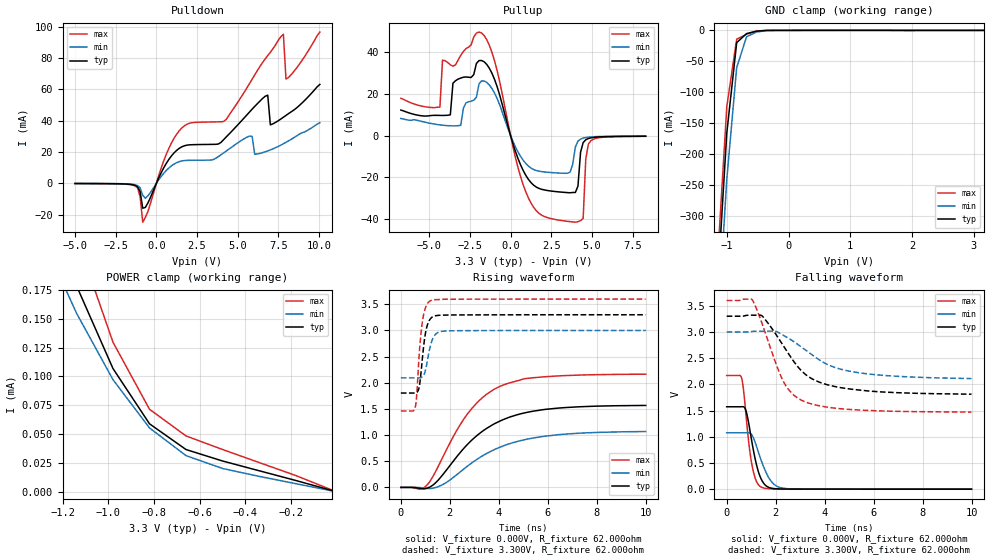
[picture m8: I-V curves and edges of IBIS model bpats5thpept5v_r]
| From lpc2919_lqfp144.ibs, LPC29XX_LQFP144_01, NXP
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| |   Rev 0.20 IBIS Model Design Automation Generation   |
| |   N O N - S I L I C O N   C O R R E L A T E D   |
| |   This IBIS [Model] is pre-Beta tactical support   |
| |  Note: this IBIS [Model] contains clamp curves generated   |
| |   through simulation which should not be relied upon   |
| Pccmos14 hliolib_nlm 4.0.1
|   0.18 um 3.3V pad library
|   six level metal
|   dual oxide
|   single threshold voltage
|   nominal line mixed supply
|   parasitic extracted netlists
| Process block c14
| bpats5thpept5v
|   Bidirectional Pad 3v3
|   3state Output
|   Plain Input
|   5ns Slew Rate control
|   CMOS
|   Programmable between
|   - (p1=0, p2=1) plain input
|   - (p1=0, p2=0) with Pull Up
|   - (p1=1, p2=1) with Pull Down
|   - (p1=1, p2=0) with Repeater
|   Characterized at Core 1.8V and I/O 3.3V
| Repeater Mode (p1=1, p2=0)
[Model]   bpats5thpept5v_r | of bpats5thpept5v
Model_type   I/O
Polarity   Non-Inverting
Enable   Active-Low
|  Reciever Thresholds
Vinl   = 0.99V
Vinh   = 2.31V
| AC Test Load Conditions
Vref   = 0
Cref   = 1.2e-11
Rref   = 1000000000
Vmeas   = 1.65
| [Process Range]   typical   min   max
| C_comp edge width   400.000ps   400.000ps   400.000ps
| C_comp Tstrobe   40.000fs   40.000fs   40.000fs
C_comp   2.536pF   2.398pF   2.677pF
[Temperature Range]   25   125   -40
[Voltage Range]   3.30V   3.00V   3.60V
[GND Clamp Reference]   0.00V   0.00V   0.00V
[Pulldown Reference]   0.00V   0.00V   0.00V
[POWER Clamp Reference]   3.30V   3.00V   3.60V
[Pullup Reference]   3.30V   3.00V   3.60V
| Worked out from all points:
|   slope of the pulldown table from 0 to 0.495 V, typ, clamps not added: 46.5 ohm
|   slope of the pullup table from 0 to 0.495 V, typ, clamps not added: 41.9 ohm
|   GND clamp passes 1 mA (typ) near -0.48 V on its own axis
|   POWER clamp passes 1 mA (typ) near -2.29 V on its own axis
|   rising waveform, V_fixture 0.000V, R_fixture 62.000ohm: 20-80 % time 2.15ns typ, 2.37ns min, 1.81ns max; typ from 0 V to 1.57 V
|   falling waveform, V_fixture 0.000V, R_fixture 62.000ohm: 20-80 % time 409ps typ, 536ps min, 320ps max; typ from 1.57 V to 0 V
|   rising waveform, V_fixture 3.300V, R_fixture 62.000ohm: 20-80 % time 225ps typ, 261ps min, 216ps max; typ from 1.8 V to 3.3 V
|   falling waveform, V_fixture 3.300V, R_fixture 62.000ohm: 20-80 % time 1.53ns typ, 1.95ns min, 1.1ns max; typ from 3.3 V to 1.81 V
[GND Clamp]
| ref voltage   0.00V   0.00V   0.00V
|   Voltage   I(typ)   I(min)   I(max)
-5V       -7.933A    -7.953A    -7.929A
-1.16V    -429.6mA   -501mA     -389.4mA
-1V       -166.1mA   -240.8mA   -123.1mA
-840mV    -19.83mA   -60.19mA   -14.2mA
-680mV    -5.242mA   -10.29mA   -6.179mA
-520mV    -1.328mA   -2.709mA   -859.7uA
-200mV    -17.4uA    -19.96uA   -26.89uA
3.16V     -7.353uA   6.327uA    -29.63uA
[Power Clamp]   | Vtable = Vcc - Vpad
| ref voltage   3.30V   3.00V   3.60V
|   Voltage   I(typ)   I(min)   I(max)
-6.74V    8.239mA    4.142mA    14.64mA
-1.3V     267.9uA    224.8uA    334.3uA
-1.14V    178.7uA    154.9uA    220.9uA
-980mV    106.8uA    97.21uA    129.7uA
-820mV    58.96uA    55.39uA    71.57uA
-660mV    36.65uA    31.38uA    48.44uA
-500mV    26.73uA    20.24uA    36.7uA
-180mV    9.891uA    7.111uA    14.19uA
-20mV     1.102uA    817.7nA    1.531uA
[Pulldown]
| ref voltage   0.00V   0.00V   0.00V
|   Voltage   I(typ)   I(min)   I(max)
-5V       -187.5uA   -145.8uA   -211.8uA
-1.32V    -1.32mA    -939.5uA   -1.723mA
-840mV    -15.95mA   -7.735mA   -24.89mA
1.56V     23.24mA    14.24mA    35.28mA
4.28V     29.46mA    20.48mA    40.61mA
5.72V     45.48mA    30.13mA    63.63mA
6.84V     56.23mA    20.64mA    81.58mA
7V        37.28mA    21.27mA    83.66mA
7.8V      42.14mA    25.2mA     95.19mA
7.96V     43.32mA    26.11mA    66.52mA
8.12V     44.49mA    27.07mA    67.59mA
10.04V    63.09mA    38.66mA    96.53mA
[Pullup]   | Vtable = Vcc - Vpad
| ref voltage   3.30V   3.00V   3.60V
|   Voltage   I(typ)   I(min)   I(max)
-6.74V    12.27mA    8.208mA    17.93mA
-4.34V    9.688mA    5.132mA    13.69mA
-4.18V    9.676mA    4.983mA    36.31mA
-3.06V    27.66mA    4.956mA    38.56mA
-1.78V    36.09mA    26.29mA    49.34mA
940mV     -19.18mA   -13.46mA   -27.14mA
3.02V     -27.13mA   -18.05mA   -40.73mA
3.98V     -27.37mA   -5.511mA   -41.66mA
4.46V     -3.361mA   -1.235mA   -39.89mA
4.62V     -2.02mA    -961.6uA   -11.27mA
4.94V     -1.105mA   -662.3uA   -2.418mA
8.3V      -310.5uA   -276.1uA   -365.1uA
[Ramp]
R_load   = 62.000ohm
|   dV/dt(typ)   dV/dt(min)   dV/dt(max)
dV/dt_r   719.308mV/2.210ns   482.040mV/2.365ns   1.047V/2.045ns
dV/dt_f   673.548mV/1.570ns   397.074mV/1.940ns   1.036V/1.245ns
[Rising Waveform]  | cubic spline decimation from 2001 points
V_fixture   = 0.000V
R_fixture   = 62.000ohm
|   Time   V(typ)   V(min)   V(max)
0s        2.367nV    410nV      1.239nV
765ps     -17.12mV   -3.17mV    -33.53mV
1.06ns    -16.24mV   -17.53mV   40.72mV
1.715ns   244.7mV    54.8mV     580.6mV
2.705ns   814.6mV    400.7mV    1.394V
3.305ns   1.064V     595.3mV    1.705V
4.07ns    1.273V     773.1mV    1.936V
4.995ns   1.418V     905.7mV    2.071V
5.89ns    1.491V     979.4mV    2.115V
10ns      1.567V     1.068V     2.164V
[Falling Waveform]  | cubic spline decimation from 2001 points
V_fixture   = 0.000V
R_fixture   = 62.000ohm
|   Time   V(typ)   V(min)   V(max)
0s        1.572V     1.075V     2.168V
605ps     1.573V     1.075V     2.128V
680ps     1.573V     1.075V     1.924V
790ps     1.493V     1.076V     1.41V
1.025ns   914.9mV    1.036V     480.1mV
1.21ns    480.2mV    828.5mV    153mV
1.44ns    165.2mV    509.9mV    33.46mV
1.875ns   15.01mV    118.9mV    4.852mV
2.4ns     2.684mV    12.88mV    1.534mV
10ns      49.4uV     117.8uV    22.88uV
[Rising Waveform]  | cubic spline decimation from 2001 points
V_fixture   = 3.300V
V_fixture_min = 3.000V
V_fixture_max = 3.600V
R_fixture   = 62.000ohm
|   Time   V(typ)   V(min)   V(max)
0s        1.804V     2.094V     1.461V
590ps     1.804V     2.094V     1.537V
640ps     1.811V     2.094V     1.714V
755ps     1.932V     2.094V     2.583V
880ps     2.466V     2.115V     3.165V
1.035ns   3.018V     2.302V     3.469V
1.235ns   3.238V     2.754V     3.574V
1.44ns    3.283V     2.937V     3.589V
1.815ns   3.294V     2.989V     3.596V
10ns      3.3V       3V         3.6V
[Falling Waveform]  | cubic spline decimation from 2001 points
V_fixture   = 3.300V
V_fixture_min = 3.000V
V_fixture_max = 3.600V
R_fixture   = 62.000ohm
|   Time   V(typ)   V(min)   V(max)
0s        3.3V       3V         3.6V
1.04ns    3.32V      3.009V     3.616V
1.45ns    3.304V     3.014V     3.152V
2.045ns   2.93V      3.004V     2.354V
2.325ns   2.728V     2.933V     2.048V
2.68ns    2.477V     2.833V     1.821V
3.07ns    2.251V     2.706V     1.693V
3.76ns    2.046V     2.474V     1.593V
4.99ns    1.914V     2.253V     1.522V
10ns      1.812V     2.11V      1.471V
